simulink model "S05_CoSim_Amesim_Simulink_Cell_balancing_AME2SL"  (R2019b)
settings: Solver=ode23s  StartTime=0  StopTime=10000  FixedStep=0.01  RelTol=1e-3  EnableMultiTasking=on
undefined symbols (not defined in the file): S05_CoSim_Amesim_Simulink_Cell_balancing_AME2SL_
libraries: simulink x1
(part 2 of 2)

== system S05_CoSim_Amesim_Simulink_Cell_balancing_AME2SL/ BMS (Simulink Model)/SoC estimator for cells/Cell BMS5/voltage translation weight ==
  I : Inport
  1-D Lookup Table : Lookup_n-D  NumberOfTableDimensions=1  BreakpointsForDimension1=[-0.6,-0.5,-0.1,0,0.1,0.5,0.6]  Table=[0,0,0.2,1,0.2,0,0]  InternalRulePriority=Speed  RndMeth=Simplest
  Add3 : Sum
  Gain2 : Gain  Gain=1/42
  Gain3 : Gain  Gain=0.5
  Transfer Fcn1 : TransferFcn  Denominator=[20*20*20 3*20*20 3*20 1]
  abs : Fcn  Expr=abs(u(1))
  VTweight : Outport
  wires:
  abs/1 -> Transfer Fcn1/1, Add3/1
  Gain2/1 -> abs/1  "Crate"
  Transfer Fcn1/1 -> Add3/2
  Add3/1 -> Gain3/1
  Gain3/1 -> 1-D Lookup Table/1
  I/1 -> Gain2/1
  1-D Lookup Table/1 -> VTweight/1

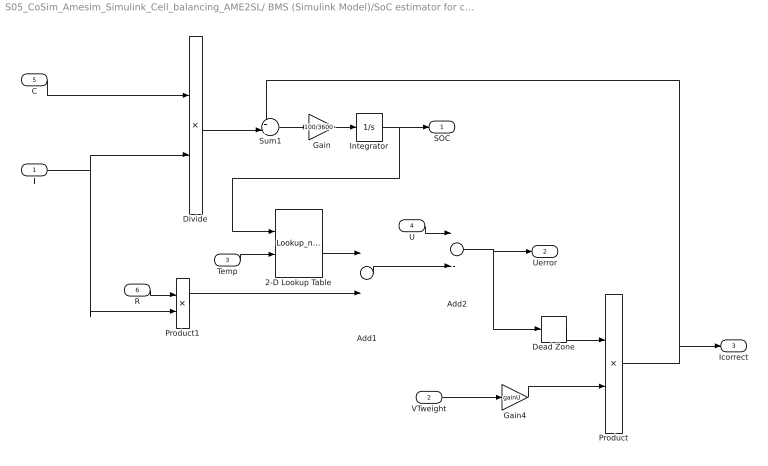
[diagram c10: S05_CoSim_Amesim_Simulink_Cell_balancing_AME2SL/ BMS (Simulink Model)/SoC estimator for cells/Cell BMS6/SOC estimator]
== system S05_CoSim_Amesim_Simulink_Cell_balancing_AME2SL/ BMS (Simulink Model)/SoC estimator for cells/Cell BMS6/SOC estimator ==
  I : Inport
  VTweight : Inport  Port=2
  Temp : Inport  Port=3
  U : Inport  Port=4
  C : Inport  Port=5
  R : Inport  Port=6
  2-D Lookup Table : Lookup_n-D  BreakpointsForDimension1=[0, 5, 10, 15, 20, 25, 30, 35, 40, 45, 50, 55, 60, 65, 70, 75, 80, 85, 90, 95, 100]  BreakpointsForDimension2=[0.00, 23.00, 40.00]  Table=[3.00912, 3.025112, 3.036932; 3.332236, 3.339581, 3.34501; 3.459481, 3.463587, 3.466622; 3.495249, 3.49837, 3.500677; 3.531047, 3.53332, 3.535; 3.560502, 3.562569, 3.564097; 3.588662, 3.589579, 3.590256; 3.62715, 3.625996, 3.625143; 3.648255, 3.64543, 3.643341; 3.66652, 3.663455, 3.66119; 3.685242, 3.681938, 3.679495; 3.70967, 3.706246, 3.703715; 3.738426, 3.735163, 3.732751; 3.780458, 3.777286, 3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  InternalRulePriority=Speed  RndMeth=Simplest
  Add1 : Sum
  Add2 : Sum  Inputs=+-
  Dead Zone : DeadZone  LowerValue=-0.005  UpperValue=0.005
  Divide : Product  Inputs=/*
  Gain : Gain  Gain=100/3600
  Gain4 : Gain  Gain=gainU
  Integrator : Integrator  InitialCondition=SOC_init
  Product : Product
  Product1 : Product
  Sum1 : Sum  Inputs=++|
  SOC : Outport
  Uerror : Outport  Port=2
  Icorrect : Outport  Port=3
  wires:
  Integrator/1 -> SOC/1, 2-D Lookup Table/1
  Gain/1 -> Integrator/1
  Sum1/1 -> Gain/1
  Add2/1 -> Uerror/1, Dead Zone/1
  Temp/1 -> 2-D Lookup Table/2
  C/1 -> Divide/1
  Divide/1 -> Sum1/2
  Gain4/1 -> Product/2
  R/1 -> Product1/1
  2-D Lookup Table/1 -> Add1/1
  Add1/1 -> Add2/2
  U/1 -> Add2/1
  Product1/1 -> Add1/2
  I/1 -> Divide/2, Product1/2
  Dead Zone/1 -> Product/1
  Product/1 -> Icorrect/1, Sum1/1
  VTweight/1 -> Gain4/1

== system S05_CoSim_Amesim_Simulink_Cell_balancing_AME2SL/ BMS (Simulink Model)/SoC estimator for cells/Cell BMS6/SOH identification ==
  I : Inport
  VTweight : Inport  Port=2
  Urerror : Inport  Port=3
  Icorrect : Inport  Port=4
  Cnom : Constant  Value=42
  Divide : Product  Inputs=**
  Divide1 : Product  Inputs=**
  Integrator3 : Integrator
  Integrator6 : Integrator
  Math Function : Math
  Math Function1 : Math
  Rnom : Constant  Value=0.0022
  Subsystem : Subsystem
  Subsystem6 : Subsystem
  C : Outport
  R : Outport  Port=2
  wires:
  I/1 -> Subsystem6/1(I), Subsystem/1(I)
  Rnom/1 -> Divide1/1
  Divide1/1 -> R/1
  Divide/1 -> C/1
  Subsystem6/1(dCcoef) -> Integrator6/1
  Integrator6/1 -> Math Function/1
  Icorrect/1 -> Subsystem6/3(Icorrect)
  Cnom/1 -> Divide/1
  Urerror/1 -> Subsystem/2(Uerror)
  Subsystem/1(dRcoef) -> Integrator3/1
  Integrator3/1 -> Math Function1/1
  VTweight/1 -> Subsystem6/2(VTweight)
  Math Function/1 -> Divide/2
  Math Function1/1 -> Divide1/2

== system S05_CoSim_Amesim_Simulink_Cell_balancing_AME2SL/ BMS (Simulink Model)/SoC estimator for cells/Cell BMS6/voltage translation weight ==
  I : Inport
  1-D Lookup Table : Lookup_n-D  NumberOfTableDimensions=1  BreakpointsForDimension1=[-0.6,-0.5,-0.1,0,0.1,0.5,0.6]  Table=[0,0,0.2,1,0.2,0,0]  InternalRulePriority=Speed  RndMeth=Simplest
  Add3 : Sum
  Gain2 : Gain  Gain=1/42
  Gain3 : Gain  Gain=0.5
  Transfer Fcn1 : TransferFcn  Denominator=[20*20*20 3*20*20 3*20 1]
  abs : Fcn  Expr=abs(u(1))
  VTweight : Outport
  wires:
  abs/1 -> Transfer Fcn1/1, Add3/1
  Gain2/1 -> abs/1  "Crate"
  Transfer Fcn1/1 -> Add3/2
  Add3/1 -> Gain3/1
  Gain3/1 -> 1-D Lookup Table/1
  I/1 -> Gain2/1
  1-D Lookup Table/1 -> VTweight/1

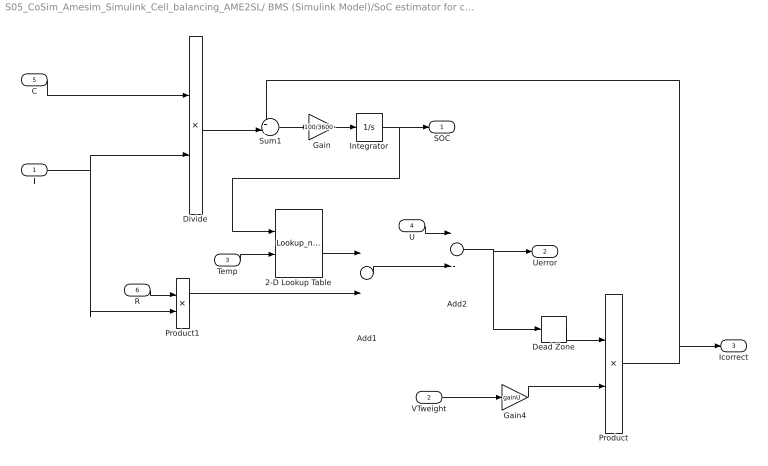
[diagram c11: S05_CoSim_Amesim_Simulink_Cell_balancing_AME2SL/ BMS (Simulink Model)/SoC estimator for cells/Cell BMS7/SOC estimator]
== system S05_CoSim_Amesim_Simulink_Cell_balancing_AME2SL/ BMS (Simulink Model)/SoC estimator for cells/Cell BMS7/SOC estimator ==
  I : Inport
  VTweight : Inport  Port=2
  Temp : Inport  Port=3
  U : Inport  Port=4
  C : Inport  Port=5
  R : Inport  Port=6
  2-D Lookup Table : Lookup_n-D  BreakpointsForDimension1=[0, 5, 10, 15, 20, 25, 30, 35, 40, 45, 50, 55, 60, 65, 70, 75, 80, 85, 90, 95, 100]  BreakpointsForDimension2=[0.00, 23.00, 40.00]  Table=[3.00912, 3.025112, 3.036932; 3.332236, 3.339581, 3.34501; 3.459481, 3.463587, 3.466622; 3.495249, 3.49837, 3.500677; 3.531047, 3.53332, 3.535; 3.560502, 3.562569, 3.564097; 3.588662, 3.589579, 3.590256; 3.62715, 3.625996, 3.625143; 3.648255, 3.64543, 3.643341; 3.66652, 3.663455, 3.66119; 3.685242, 3.681938, 3.679495; 3.70967, 3.706246, 3.703715; 3.738426, 3.735163, 3.732751; 3.780458, 3.777286, 3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  InternalRulePriority=Speed  RndMeth=Simplest
  Add1 : Sum
  Add2 : Sum  Inputs=+-
  Dead Zone : DeadZone  LowerValue=-0.005  UpperValue=0.005
  Divide : Product  Inputs=/*
  Gain : Gain  Gain=100/3600
  Gain4 : Gain  Gain=gainU
  Integrator : Integrator  InitialCondition=SOC_init
  Product : Product
  Product1 : Product
  Sum1 : Sum  Inputs=++|
  SOC : Outport
  Uerror : Outport  Port=2
  Icorrect : Outport  Port=3
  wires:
  Integrator/1 -> SOC/1, 2-D Lookup Table/1
  Gain/1 -> Integrator/1
  Sum1/1 -> Gain/1
  Add2/1 -> Uerror/1, Dead Zone/1
  Temp/1 -> 2-D Lookup Table/2
  C/1 -> Divide/1
  Divide/1 -> Sum1/2
  Gain4/1 -> Product/2
  R/1 -> Product1/1
  2-D Lookup Table/1 -> Add1/1
  Add1/1 -> Add2/2
  U/1 -> Add2/1
  Product1/1 -> Add1/2
  I/1 -> Divide/2, Product1/2
  Dead Zone/1 -> Product/1
  Product/1 -> Icorrect/1, Sum1/1
  VTweight/1 -> Gain4/1

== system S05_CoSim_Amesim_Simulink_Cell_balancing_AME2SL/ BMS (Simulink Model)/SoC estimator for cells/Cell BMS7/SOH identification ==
  I : Inport
  VTweight : Inport  Port=2
  Urerror : Inport  Port=3
  Icorrect : Inport  Port=4
  Cnom : Constant  Value=42
  Divide : Product  Inputs=**
  Divide1 : Product  Inputs=**
  Integrator3 : Integrator
  Integrator6 : Integrator
  Math Function : Math
  Math Function1 : Math
  Rnom : Constant  Value=0.0022
  Subsystem : Subsystem
  Subsystem6 : Subsystem
  C : Outport
  R : Outport  Port=2
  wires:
  I/1 -> Subsystem6/1(I), Subsystem/1(I)
  Rnom/1 -> Divide1/1
  Divide1/1 -> R/1
  Divide/1 -> C/1
  Subsystem6/1(dCcoef) -> Integrator6/1
  Integrator6/1 -> Math Function/1
  Icorrect/1 -> Subsystem6/3(Icorrect)
  Cnom/1 -> Divide/1
  Urerror/1 -> Subsystem/2(Uerror)
  Subsystem/1(dRcoef) -> Integrator3/1
  Integrator3/1 -> Math Function1/1
  VTweight/1 -> Subsystem6/2(VTweight)
  Math Function/1 -> Divide/2
  Math Function1/1 -> Divide1/2

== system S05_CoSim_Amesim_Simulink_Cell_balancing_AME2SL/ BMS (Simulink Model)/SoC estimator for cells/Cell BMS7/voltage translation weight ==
  I : Inport
  1-D Lookup Table : Lookup_n-D  NumberOfTableDimensions=1  BreakpointsForDimension1=[-0.6,-0.5,-0.1,0,0.1,0.5,0.6]  Table=[0,0,0.2,1,0.2,0,0]  InternalRulePriority=Speed  RndMeth=Simplest
  Add3 : Sum
  Gain2 : Gain  Gain=1/42
  Gain3 : Gain  Gain=0.5
  Transfer Fcn1 : TransferFcn  Denominator=[20*20*20 3*20*20 3*20 1]
  abs : Fcn  Expr=abs(u(1))
  VTweight : Outport
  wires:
  abs/1 -> Transfer Fcn1/1, Add3/1
  Gain2/1 -> abs/1  "Crate"
  Transfer Fcn1/1 -> Add3/2
  Add3/1 -> Gain3/1
  Gain3/1 -> 1-D Lookup Table/1
  I/1 -> Gain2/1
  1-D Lookup Table/1 -> VTweight/1

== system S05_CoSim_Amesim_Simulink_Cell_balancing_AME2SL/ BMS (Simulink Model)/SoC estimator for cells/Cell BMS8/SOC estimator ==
  I : Inport
  VTweight : Inport  Port=2
  Temp : Inport  Port=3
  U : Inport  Port=4
  C : Inport  Port=5
  R : Inport  Port=6
  2-D Lookup Table : Lookup_n-D  BreakpointsForDimension1=[0, 5, 10, 15, 20, 25, 30, 35, 40, 45, 50, 55, 60, 65, 70, 75, 80, 85, 90, 95, 100]  BreakpointsForDimension2=[0.00, 23.00, 40.00]  Table=[3.00912, 3.025112, 3.036932; 3.332236, 3.339581, 3.34501; 3.459481, 3.463587, 3.466622; 3.495249, 3.49837, 3.500677; 3.531047, 3.53332, 3.535; 3.560502, 3.562569, 3.564097; 3.588662, 3.589579, 3.590256; 3.62715, 3.625996, 3.625143; 3.648255, 3.64543, 3.643341; 3.66652, 3.663455, 3.66119; 3.685242, 3.681938, 3.679495; 3.70967, 3.706246, 3.703715; 3.738426, 3.735163, 3.732751; 3.780458, 3.777286, 3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  InternalRulePriority=Speed  RndMeth=Simplest
  Add1 : Sum
  Add2 : Sum  Inputs=+-
  Dead Zone : DeadZone  LowerValue=-0.005  UpperValue=0.005
  Divide : Product  Inputs=/*
  Gain : Gain  Gain=100/3600
  Gain4 : Gain  Gain=gainU
  Integrator : Integrator  InitialCondition=SOC_init
  Product : Product
  Product1 : Product
  Sum1 : Sum  Inputs=++|
  SOC : Outport
  Uerror : Outport  Port=2
  Icorrect : Outport  Port=3
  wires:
  Integrator/1 -> SOC/1, 2-D Lookup Table/1
  Gain/1 -> Integrator/1
  Sum1/1 -> Gain/1
  Add2/1 -> Uerror/1, Dead Zone/1
  Temp/1 -> 2-D Lookup Table/2
  C/1 -> Divide/1
  Divide/1 -> Sum1/2
  Gain4/1 -> Product/2
  R/1 -> Product1/1
  2-D Lookup Table/1 -> Add1/1
  Add1/1 -> Add2/2
  U/1 -> Add2/1
  Product1/1 -> Add1/2
  I/1 -> Divide/2, Product1/2
  Dead Zone/1 -> Product/1
  Product/1 -> Icorrect/1, Sum1/1
  VTweight/1 -> Gain4/1

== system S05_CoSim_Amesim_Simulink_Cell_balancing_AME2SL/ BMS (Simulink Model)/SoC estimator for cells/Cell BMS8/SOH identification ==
  I : Inport
  VTweight : Inport  Port=2
  Urerror : Inport  Port=3
  Icorrect : Inport  Port=4
  Cnom : Constant  Value=42
  Divide : Product  Inputs=**
  Divide1 : Product  Inputs=**
  Integrator3 : Integrator
  Integrator6 : Integrator
  Math Function : Math
  Math Function1 : Math
  Rnom : Constant  Value=0.0022
  Subsystem : Subsystem
  Subsystem6 : Subsystem
  C : Outport
  R : Outport  Port=2
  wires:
  I/1 -> Subsystem6/1(I), Subsystem/1(I)
  Rnom/1 -> Divide1/1
  Divide1/1 -> R/1
  Divide/1 -> C/1
  Subsystem6/1(dCcoef) -> Integrator6/1
  Integrator6/1 -> Math Function/1
  Icorrect/1 -> Subsystem6/3(Icorrect)
  Cnom/1 -> Divide/1
  Urerror/1 -> Subsystem/2(Uerror)
  Subsystem/1(dRcoef) -> Integrator3/1
  Integrator3/1 -> Math Function1/1
  VTweight/1 -> Subsystem6/2(VTweight)
  Math Function/1 -> Divide/2
  Math Function1/1 -> Divide1/2

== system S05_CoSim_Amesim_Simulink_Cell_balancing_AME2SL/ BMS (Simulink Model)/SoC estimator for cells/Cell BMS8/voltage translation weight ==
  I : Inport
  1-D Lookup Table : Lookup_n-D  NumberOfTableDimensions=1  BreakpointsForDimension1=[-0.6,-0.5,-0.1,0,0.1,0.5,0.6]  Table=[0,0,0.2,1,0.2,0,0]  InternalRulePriority=Speed  RndMeth=Simplest
  Add3 : Sum
  Gain2 : Gain  Gain=1/42
  Gain3 : Gain  Gain=0.5
  Transfer Fcn1 : TransferFcn  Denominator=[20*20*20 3*20*20 3*20 1]
  abs : Fcn  Expr=abs(u(1))
  VTweight : Outport
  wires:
  abs/1 -> Transfer Fcn1/1, Add3/1
  Gain2/1 -> abs/1  "Crate"
  Transfer Fcn1/1 -> Add3/2
  Add3/1 -> Gain3/1
  Gain3/1 -> 1-D Lookup Table/1
  I/1 -> Gain2/1
  1-D Lookup Table/1 -> VTweight/1

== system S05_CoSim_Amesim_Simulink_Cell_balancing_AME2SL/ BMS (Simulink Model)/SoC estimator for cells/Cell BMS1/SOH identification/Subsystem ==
  I : Inport
  Uerror : Inport  Port=2
  Gain : Gain  Gain=0.0005
  Gain1 : Gain  Gain=1/42
  Product : Product
  Sqrt : Sqrt  Operator=signedSqrt
  Transfer Fcn1 : TransferFcn  Numerator=[300 0]  Denominator=[300 1]
  Transfer Fcn4 : TransferFcn  Denominator=[20*20*20 3*20*20 3*20 1]
  dRcoef : Outport
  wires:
  Gain/1 -> dRcoef/1
  Gain1/1 -> Product/1
  Sqrt/1 -> Gain/1
  I/1 -> Gain1/1
  Transfer Fcn4/1 -> Transfer Fcn1/1
  Uerror/1 -> Product/2
  Product/1 -> Transfer Fcn4/1
  Transfer Fcn1/1 -> Sqrt/1

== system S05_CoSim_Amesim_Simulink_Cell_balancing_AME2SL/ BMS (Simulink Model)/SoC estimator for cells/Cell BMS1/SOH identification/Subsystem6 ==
  I : Inport
  VTweight : Inport  Port=2
  Icorrect : Inport  Port=3
  DSOC : Scope
  Gain : Gain  Gain=0.0004
  Gain1 : Gain  Gain=-1
  Gain2 : Gain  Gain=1/42
  Gain3 : Gain  Gain=1/42
  Gain4 : Gain  Gain=100/3600
  Gain5 : Gain  Gain=0.1
  Icor : Scope
  Integrator : Integrator
  Product : Product
  Product1 : Product
  Sum : Sum  Inputs=|+-
  Transfer Fcn1 : TransferFcn  Denominator=[120*120*120 3*120*120 3*120 1]
  VT : Scope
  dC_dt : Scope
  dCcoef : Outport
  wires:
  Product/1 -> Gain1/1
  Gain/1 -> dCcoef/1
  Icorrect/1 -> Gain3/1
  I/1 -> Gain2/1
  Sum/1 -> Gain4/1
  Integrator/1 -> DSOC/1, Product/1, Product1/1
  Gain2/1 -> Sum/1
  Gain3/1 -> Icor/1, Product/2
  Gain4/1 -> Integrator/1
  Product1/1 -> Gain5/1
  VTweight/1 -> Transfer Fcn1/1, VT/1
  Gain5/1 -> Sum/2
  Gain1/1 -> dC_dt/1, Gain/1
  Transfer Fcn1/1 -> Product1/2

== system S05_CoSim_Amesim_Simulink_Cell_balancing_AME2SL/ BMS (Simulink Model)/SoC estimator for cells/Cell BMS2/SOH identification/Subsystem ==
  I : Inport
  Uerror : Inport  Port=2
  Gain : Gain  Gain=0.0005
  Gain1 : Gain  Gain=1/42
  Product : Product
  Sqrt : Sqrt  Operator=signedSqrt
  Transfer Fcn1 : TransferFcn  Numerator=[300 0]  Denominator=[300 1]
  Transfer Fcn4 : TransferFcn  Denominator=[20*20*20 3*20*20 3*20 1]
  dRcoef : Outport
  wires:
  Gain/1 -> dRcoef/1
  Gain1/1 -> Product/1
  Sqrt/1 -> Gain/1
  I/1 -> Gain1/1
  Transfer Fcn4/1 -> Transfer Fcn1/1
  Uerror/1 -> Product/2
  Product/1 -> Transfer Fcn4/1
  Transfer Fcn1/1 -> Sqrt/1

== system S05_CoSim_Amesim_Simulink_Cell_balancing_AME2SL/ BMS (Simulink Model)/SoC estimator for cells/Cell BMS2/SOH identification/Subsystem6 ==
  I : Inport
  VTweight : Inport  Port=2
  Icorrect : Inport  Port=3
  DSOC : Scope
  Gain : Gain  Gain=0.0004
  Gain1 : Gain  Gain=-1
  Gain2 : Gain  Gain=1/42
  Gain3 : Gain  Gain=1/42
  Gain4 : Gain  Gain=100/3600
  Gain5 : Gain  Gain=0.1
  Icor : Scope
  Integrator : Integrator
  Product : Product
  Product1 : Product
  Sum : Sum  Inputs=|+-
  Transfer Fcn1 : TransferFcn  Denominator=[120*120*120 3*120*120 3*120 1]
  VT : Scope
  dC_dt : Scope
  dCcoef : Outport
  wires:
  Product/1 -> Gain1/1
  Gain/1 -> dCcoef/1
  Icorrect/1 -> Gain3/1
  I/1 -> Gain2/1
  Sum/1 -> Gain4/1
  Integrator/1 -> DSOC/1, Product/1, Product1/1
  Gain2/1 -> Sum/1
  Gain3/1 -> Icor/1, Product/2
  Gain4/1 -> Integrator/1
  Product1/1 -> Gain5/1
  VTweight/1 -> Transfer Fcn1/1, VT/1
  Gain5/1 -> Sum/2
  Gain1/1 -> dC_dt/1, Gain/1
  Transfer Fcn1/1 -> Product1/2

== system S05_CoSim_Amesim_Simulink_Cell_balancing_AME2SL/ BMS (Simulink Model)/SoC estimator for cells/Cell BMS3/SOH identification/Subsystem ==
  I : Inport
  Uerror : Inport  Port=2
  Gain : Gain  Gain=0.0005
  Gain1 : Gain  Gain=1/42
  Product : Product
  Sqrt : Sqrt  Operator=signedSqrt
  Transfer Fcn1 : TransferFcn  Numerator=[300 0]  Denominator=[300 1]
  Transfer Fcn4 : TransferFcn  Denominator=[20*20*20 3*20*20 3*20 1]
  dRcoef : Outport
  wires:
  Gain/1 -> dRcoef/1
  Gain1/1 -> Product/1
  Sqrt/1 -> Gain/1
  I/1 -> Gain1/1
  Transfer Fcn4/1 -> Transfer Fcn1/1
  Uerror/1 -> Product/2
  Product/1 -> Transfer Fcn4/1
  Transfer Fcn1/1 -> Sqrt/1

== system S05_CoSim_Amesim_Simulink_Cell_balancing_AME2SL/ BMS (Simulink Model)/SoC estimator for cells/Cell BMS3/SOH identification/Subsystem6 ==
  I : Inport
  VTweight : Inport  Port=2
  Icorrect : Inport  Port=3
  DSOC : Scope
  Gain : Gain  Gain=0.0004
  Gain1 : Gain  Gain=-1
  Gain2 : Gain  Gain=1/42
  Gain3 : Gain  Gain=1/42
  Gain4 : Gain  Gain=100/3600
  Gain5 : Gain  Gain=0.1
  Icor : Scope
  Integrator : Integrator
  Product : Product
  Product1 : Product
  Sum : Sum  Inputs=|+-
  Transfer Fcn1 : TransferFcn  Denominator=[120*120*120 3*120*120 3*120 1]
  VT : Scope
  dC_dt : Scope
  dCcoef : Outport
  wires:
  Product/1 -> Gain1/1
  Gain/1 -> dCcoef/1
  Icorrect/1 -> Gain3/1
  I/1 -> Gain2/1
  Sum/1 -> Gain4/1
  Integrator/1 -> DSOC/1, Product/1, Product1/1
  Gain2/1 -> Sum/1
  Gain3/1 -> Icor/1, Product/2
  Gain4/1 -> Integrator/1
  Product1/1 -> Gain5/1
  VTweight/1 -> Transfer Fcn1/1, VT/1
  Gain5/1 -> Sum/2
  Gain1/1 -> dC_dt/1, Gain/1
  Transfer Fcn1/1 -> Product1/2

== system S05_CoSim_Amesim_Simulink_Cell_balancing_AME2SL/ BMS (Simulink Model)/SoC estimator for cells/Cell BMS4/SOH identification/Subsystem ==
  I : Inport
  Uerror : Inport  Port=2
  Gain : Gain  Gain=0.0005
  Gain1 : Gain  Gain=1/42
  Product : Product
  Sqrt : Sqrt  Operator=signedSqrt
  Transfer Fcn1 : TransferFcn  Numerator=[300 0]  Denominator=[300 1]
  Transfer Fcn4 : TransferFcn  Denominator=[20*20*20 3*20*20 3*20 1]
  dRcoef : Outport
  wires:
  Gain/1 -> dRcoef/1
  Gain1/1 -> Product/1
  Sqrt/1 -> Gain/1
  I/1 -> Gain1/1
  Transfer Fcn4/1 -> Transfer Fcn1/1
  Uerror/1 -> Product/2
  Product/1 -> Transfer Fcn4/1
  Transfer Fcn1/1 -> Sqrt/1

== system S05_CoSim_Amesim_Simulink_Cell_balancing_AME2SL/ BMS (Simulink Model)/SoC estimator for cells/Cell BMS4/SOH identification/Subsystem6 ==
  I : Inport
  VTweight : Inport  Port=2
  Icorrect : Inport  Port=3
  DSOC : Scope
  Gain : Gain  Gain=0.0004
  Gain1 : Gain  Gain=-1
  Gain2 : Gain  Gain=1/42
  Gain3 : Gain  Gain=1/42
  Gain4 : Gain  Gain=100/3600
  Gain5 : Gain  Gain=0.1
  Icor : Scope
  Integrator : Integrator
  Product : Product
  Product1 : Product
  Sum : Sum  Inputs=|+-
  Transfer Fcn1 : TransferFcn  Denominator=[120*120*120 3*120*120 3*120 1]
  VT : Scope
  dC_dt : Scope
  dCcoef : Outport
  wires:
  Product/1 -> Gain1/1
  Gain/1 -> dCcoef/1
  Icorrect/1 -> Gain3/1
  I/1 -> Gain2/1
  Sum/1 -> Gain4/1
  Integrator/1 -> DSOC/1, Product/1, Product1/1
  Gain2/1 -> Sum/1
  Gain3/1 -> Icor/1, Product/2
  Gain4/1 -> Integrator/1
  Product1/1 -> Gain5/1
  VTweight/1 -> Transfer Fcn1/1, VT/1
  Gain5/1 -> Sum/2
  Gain1/1 -> dC_dt/1, Gain/1
  Transfer Fcn1/1 -> Product1/2

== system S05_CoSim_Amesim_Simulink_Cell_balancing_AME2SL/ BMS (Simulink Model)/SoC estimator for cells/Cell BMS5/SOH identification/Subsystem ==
  I : Inport
  Uerror : Inport  Port=2
  Gain : Gain  Gain=0.0005
  Gain1 : Gain  Gain=1/42
  Product : Product
  Sqrt : Sqrt  Operator=signedSqrt
  Transfer Fcn1 : TransferFcn  Numerator=[300 0]  Denominator=[300 1]
  Transfer Fcn4 : TransferFcn  Denominator=[20*20*20 3*20*20 3*20 1]
  dRcoef : Outport
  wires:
  Gain/1 -> dRcoef/1
  Gain1/1 -> Product/1
  Sqrt/1 -> Gain/1
  I/1 -> Gain1/1
  Transfer Fcn4/1 -> Transfer Fcn1/1
  Uerror/1 -> Product/2
  Product/1 -> Transfer Fcn4/1
  Transfer Fcn1/1 -> Sqrt/1

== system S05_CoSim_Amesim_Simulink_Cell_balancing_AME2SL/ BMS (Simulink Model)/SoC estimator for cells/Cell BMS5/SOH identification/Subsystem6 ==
  I : Inport
  VTweight : Inport  Port=2
  Icorrect : Inport  Port=3
  DSOC : Scope
  Gain : Gain  Gain=0.0004
  Gain1 : Gain  Gain=-1
  Gain2 : Gain  Gain=1/42
  Gain3 : Gain  Gain=1/42
  Gain4 : Gain  Gain=100/3600
  Gain5 : Gain  Gain=0.1
  Icor : Scope
  Integrator : Integrator
  Product : Product
  Product1 : Product
  Sum : Sum  Inputs=|+-
  Transfer Fcn1 : TransferFcn  Denominator=[120*120*120 3*120*120 3*120 1]
  VT : Scope
  dC_dt : Scope
  dCcoef : Outport
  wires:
  Product/1 -> Gain1/1
  Gain/1 -> dCcoef/1
  Icorrect/1 -> Gain3/1
  I/1 -> Gain2/1
  Sum/1 -> Gain4/1
  Integrator/1 -> DSOC/1, Product/1, Product1/1
  Gain2/1 -> Sum/1
  Gain3/1 -> Icor/1, Product/2
  Gain4/1 -> Integrator/1
  Product1/1 -> Gain5/1
  VTweight/1 -> Transfer Fcn1/1, VT/1
  Gain5/1 -> Sum/2
  Gain1/1 -> dC_dt/1, Gain/1
  Transfer Fcn1/1 -> Product1/2

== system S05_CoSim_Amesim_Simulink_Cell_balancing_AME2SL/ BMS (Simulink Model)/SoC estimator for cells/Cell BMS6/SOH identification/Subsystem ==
  I : Inport
  Uerror : Inport  Port=2
  Gain : Gain  Gain=0.0005
  Gain1 : Gain  Gain=1/42
  Product : Product
  Sqrt : Sqrt  Operator=signedSqrt
  Transfer Fcn1 : TransferFcn  Numerator=[300 0]  Denominator=[300 1]
  Transfer Fcn4 : TransferFcn  Denominator=[20*20*20 3*20*20 3*20 1]
  dRcoef : Outport
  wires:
  Gain/1 -> dRcoef/1
  Gain1/1 -> Product/1
  Sqrt/1 -> Gain/1
  I/1 -> Gain1/1
  Transfer Fcn4/1 -> Transfer Fcn1/1
  Uerror/1 -> Product/2
  Product/1 -> Transfer Fcn4/1
  Transfer Fcn1/1 -> Sqrt/1

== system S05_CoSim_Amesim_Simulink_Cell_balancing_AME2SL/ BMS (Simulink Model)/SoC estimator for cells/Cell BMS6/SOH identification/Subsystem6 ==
  I : Inport
  VTweight : Inport  Port=2
  Icorrect : Inport  Port=3
  DSOC : Scope
  Gain : Gain  Gain=0.0004
  Gain1 : Gain  Gain=-1
  Gain2 : Gain  Gain=1/42
  Gain3 : Gain  Gain=1/42
  Gain4 : Gain  Gain=100/3600
  Gain5 : Gain  Gain=0.1
  Icor : Scope
  Integrator : Integrator
  Product : Product
  Product1 : Product
  Sum : Sum  Inputs=|+-
  Transfer Fcn1 : TransferFcn  Denominator=[120*120*120 3*120*120 3*120 1]
  VT : Scope
  dC_dt : Scope
  dCcoef : Outport
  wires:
  Product/1 -> Gain1/1
  Gain/1 -> dCcoef/1
  Icorrect/1 -> Gain3/1
  I/1 -> Gain2/1
  Sum/1 -> Gain4/1
  Integrator/1 -> DSOC/1, Product/1, Product1/1
  Gain2/1 -> Sum/1
  Gain3/1 -> Icor/1, Product/2
  Gain4/1 -> Integrator/1
  Product1/1 -> Gain5/1
  VTweight/1 -> Transfer Fcn1/1, VT/1
  Gain5/1 -> Sum/2
  Gain1/1 -> dC_dt/1, Gain/1
  Transfer Fcn1/1 -> Product1/2

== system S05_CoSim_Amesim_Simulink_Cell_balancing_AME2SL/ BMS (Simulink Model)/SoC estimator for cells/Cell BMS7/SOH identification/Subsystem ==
  I : Inport
  Uerror : Inport  Port=2
  Gain : Gain  Gain=0.0005
  Gain1 : Gain  Gain=1/42
  Product : Product
  Sqrt : Sqrt  Operator=signedSqrt
  Transfer Fcn1 : TransferFcn  Numerator=[300 0]  Denominator=[300 1]
  Transfer Fcn4 : TransferFcn  Denominator=[20*20*20 3*20*20 3*20 1]
  dRcoef : Outport
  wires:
  Gain/1 -> dRcoef/1
  Gain1/1 -> Product/1
  Sqrt/1 -> Gain/1
  I/1 -> Gain1/1
  Transfer Fcn4/1 -> Transfer Fcn1/1
  Uerror/1 -> Product/2
  Product/1 -> Transfer Fcn4/1
  Transfer Fcn1/1 -> Sqrt/1

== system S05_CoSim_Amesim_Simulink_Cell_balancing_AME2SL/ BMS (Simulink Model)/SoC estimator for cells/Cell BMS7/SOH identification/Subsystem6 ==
  I : Inport
  VTweight : Inport  Port=2
  Icorrect : Inport  Port=3
  DSOC : Scope
  Gain : Gain  Gain=0.0004
  Gain1 : Gain  Gain=-1
  Gain2 : Gain  Gain=1/42
  Gain3 : Gain  Gain=1/42
  Gain4 : Gain  Gain=100/3600
  Gain5 : Gain  Gain=0.1
  Icor : Scope
  Integrator : Integrator
  Product : Product
  Product1 : Product
  Sum : Sum  Inputs=|+-
  Transfer Fcn1 : TransferFcn  Denominator=[120*120*120 3*120*120 3*120 1]
  VT : Scope
  dC_dt : Scope
  dCcoef : Outport
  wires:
  Product/1 -> Gain1/1
  Gain/1 -> dCcoef/1
  Icorrect/1 -> Gain3/1
  I/1 -> Gain2/1
  Sum/1 -> Gain4/1
  Integrator/1 -> DSOC/1, Product/1, Product1/1
  Gain2/1 -> Sum/1
  Gain3/1 -> Icor/1, Product/2
  Gain4/1 -> Integrator/1
  Product1/1 -> Gain5/1
  VTweight/1 -> Transfer Fcn1/1, VT/1
  Gain5/1 -> Sum/2
  Gain1/1 -> dC_dt/1, Gain/1
  Transfer Fcn1/1 -> Product1/2

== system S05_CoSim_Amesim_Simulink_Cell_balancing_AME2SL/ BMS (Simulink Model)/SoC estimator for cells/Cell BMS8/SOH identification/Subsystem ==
  I : Inport
  Uerror : Inport  Port=2
  Gain : Gain  Gain=0.0005
  Gain1 : Gain  Gain=1/42
  Product : Product
  Sqrt : Sqrt  Operator=signedSqrt
  Transfer Fcn1 : TransferFcn  Numerator=[300 0]  Denominator=[300 1]
  Transfer Fcn4 : TransferFcn  Denominator=[20*20*20 3*20*20 3*20 1]
  dRcoef : Outport
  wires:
  Gain/1 -> dRcoef/1
  Gain1/1 -> Product/1
  Sqrt/1 -> Gain/1
  I/1 -> Gain1/1
  Transfer Fcn4/1 -> Transfer Fcn1/1
  Uerror/1 -> Product/2
  Product/1 -> Transfer Fcn4/1
  Transfer Fcn1/1 -> Sqrt/1

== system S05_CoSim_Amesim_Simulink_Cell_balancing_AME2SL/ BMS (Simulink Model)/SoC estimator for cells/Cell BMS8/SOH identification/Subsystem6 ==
  I : Inport
  VTweight : Inport  Port=2
  Icorrect : Inport  Port=3
  DSOC : Scope
  Gain : Gain  Gain=0.0004
  Gain1 : Gain  Gain=-1
  Gain2 : Gain  Gain=1/42
  Gain3 : Gain  Gain=1/42
  Gain4 : Gain  Gain=100/3600
  Gain5 : Gain  Gain=0.1
  Icor : Scope
  Integrator : Integrator
  Product : Product
  Product1 : Product
  Sum : Sum  Inputs=|+-
  Transfer Fcn1 : TransferFcn  Denominator=[120*120*120 3*120*120 3*120 1]
  VT : Scope
  dC_dt : Scope
  dCcoef : Outport
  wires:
  Product/1 -> Gain1/1
  Gain/1 -> dCcoef/1
  Icorrect/1 -> Gain3/1
  I/1 -> Gain2/1
  Sum/1 -> Gain4/1
  Integrator/1 -> DSOC/1, Product/1, Product1/1
  Gain2/1 -> Sum/1
  Gain3/1 -> Icor/1, Product/2
  Gain4/1 -> Integrator/1
  Product1/1 -> Gain5/1
  VTweight/1 -> Transfer Fcn1/1, VT/1
  Gain5/1 -> Sum/2
  Gain1/1 -> dC_dt/1, Gain/1
  Transfer Fcn1/1 -> Product1/2

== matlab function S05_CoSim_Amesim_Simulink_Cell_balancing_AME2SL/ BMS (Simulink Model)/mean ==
function y = fcn(u)
%#codegen

y = mean(u);

== matlab function S05_CoSim_Amesim_Simulink_Cell_balancing_AME2SL/ BMS (Simulink Model)/Balancing decision 
based on SoCcontrol/median ==
function y = fcn(u)
%#codegen

y = median(u);

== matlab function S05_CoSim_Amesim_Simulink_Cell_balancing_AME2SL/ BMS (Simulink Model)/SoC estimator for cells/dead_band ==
function y = fcn(u)
%#codegen

y = u*(abs(u)>0.4);

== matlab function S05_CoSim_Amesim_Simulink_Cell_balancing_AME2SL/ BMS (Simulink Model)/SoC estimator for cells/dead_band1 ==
function y = fcn(u)
%#codegen

y = u*(abs(u)>0.4);

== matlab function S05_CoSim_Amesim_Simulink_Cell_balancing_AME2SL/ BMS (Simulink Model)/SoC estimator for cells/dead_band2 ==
function y = fcn(u)
%#codegen

y = u*(abs(u)>0.4);

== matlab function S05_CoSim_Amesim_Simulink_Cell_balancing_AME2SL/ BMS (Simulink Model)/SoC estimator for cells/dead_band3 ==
function y = fcn(u)
%#codegen

y = u*(abs(u)>0.4);

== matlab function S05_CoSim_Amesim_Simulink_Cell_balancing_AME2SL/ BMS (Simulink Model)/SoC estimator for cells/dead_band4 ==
function y = fcn(u)
%#codegen

y = u*(abs(u)>0.4);

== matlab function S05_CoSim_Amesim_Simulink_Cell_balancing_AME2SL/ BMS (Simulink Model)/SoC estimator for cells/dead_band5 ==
function y = fcn(u)
%#codegen

y = u*(abs(u)>0.4);

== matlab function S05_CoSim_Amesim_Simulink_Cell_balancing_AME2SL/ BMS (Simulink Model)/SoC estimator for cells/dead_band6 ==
function y = fcn(u)
%#codegen

y = u*(abs(u)>0.4);

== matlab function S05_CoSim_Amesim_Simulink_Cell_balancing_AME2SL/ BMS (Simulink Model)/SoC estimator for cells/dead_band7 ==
function y = fcn(u)
%#codegen

y = u*(abs(u)>0.4);
